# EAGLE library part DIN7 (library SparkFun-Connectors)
Mini-DIN7 Connector Through-hole MiniDIN 7 connector. Commonly used with Roomba products. Don't confuse this with DIN-6, which is commonly used on oldschool keyboards and mice. Here is the female version connector we sell at SparkFun: MiniDIN 7-Pin Connector (PRT-00696)
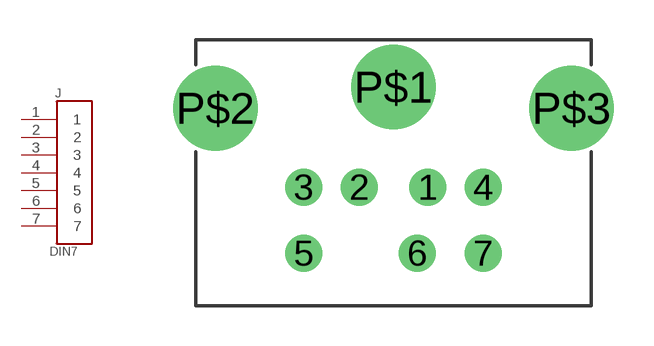
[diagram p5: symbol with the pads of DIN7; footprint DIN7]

Designator prefix J

## DIN7 (PROD_ID: CONN-08318; SF_ID: PRT-00696)  [DIN7]
1  1
2  2
3  3
4  4
5  5
6  6
7  7

## Footprint DIN7 (pad centres in mm)
miniDIN Right Angle Specifications: Pin count:7 Datasheet referenced for footprint Example device(s): DIN7
drill 0.9: 1 1.3,-3.8; 2 -1.3,-3.8; 3 -3.4,-3.8; 4 3.4,-3.8; 5 -3.4,-6.3; 6 0.9,-6.3; 7 3.4,-6.3
drill 2.2: P$1 0,0; P$2 -6.75,-0.8; P$3 6.75,-0.8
